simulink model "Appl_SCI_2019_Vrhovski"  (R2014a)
settings: Solver=ode45  StartTime=0.0  StopTime=1000  MaxStep=0.01  RelTol=1e-3
undefined symbols (not defined in the file): deg, H, kg, m, M, mm, N, rad, s, X, Y, Z
libraries: sm_lib x389, nesl_utility x69, simulink x7
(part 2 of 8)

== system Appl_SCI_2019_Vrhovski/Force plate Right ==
  Center of Presure : MATLAB Function  TreatAsAtomicUnit=on
  Donja ploca : Subsystem
  Gornja ploca : Subsystem
  Komponente senzora sile : Subsystem
  Senzori sile : Subsystem
  F : PMIOPort  Port=1  Side=Right
  B : PMIOPort  Port=2  Side=Left
  CoP_x : Outport
  CoP_y : Outport  Port=2
  Fz : Outport  Port=3
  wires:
  Komponente senzora sile/3(F1z) -> Center of Presure/1(Fz1)
  Komponente senzora sile/6(F2z) -> Center of Presure/2(Fz2)
  Komponente senzora sile/9(F3z) -> Center of Presure/3(Fz3)
  Komponente senzora sile/12(F4z) -> Center of Presure/4(Fz4)
  Center of Presure/1(CoP_x) -> CoP_x/1
  Center of Presure/2(CoP_y) -> CoP_y/1
  Center of Presure/3(F_suma) -> Fz/1
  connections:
  Senzori sile/RConn8 -- Komponente senzora sile/LConn4
  Senzori sile/RConn6 -- Komponente senzora sile/LConn3
  Komponente senzora sile/LConn2 -- Senzori sile/RConn4
  Senzori sile/RConn2 -- Komponente senzora sile/LConn1
  B/RConn1 -- Donja ploca/LConn1
  Gornja ploca/LConn3 -- Senzori sile/RConn5
  Senzori sile/RConn7 -- Gornja ploca/LConn4
  F/RConn1 -- Gornja ploca/RConn1
  Senzori sile/RConn3 -- Gornja ploca/LConn2
  Gornja ploca/LConn1 -- Senzori sile/RConn1
  Donja ploca/RConn4 -- Senzori sile/LConn4
  Donja ploca/RConn2 -- Senzori sile/LConn2
  Donja ploca/RConn3 -- Senzori sile/LConn3
  Donja ploca/RConn1 -- Senzori sile/LConn1

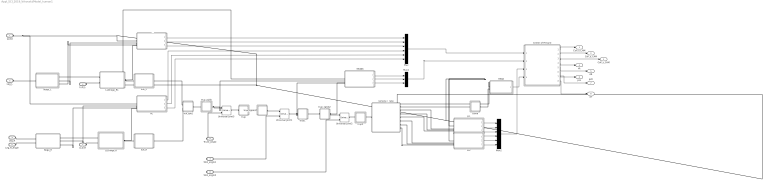
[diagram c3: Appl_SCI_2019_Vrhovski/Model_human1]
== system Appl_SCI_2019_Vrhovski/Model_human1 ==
  Center of Presure : MATLAB Function  TreatAsAtomicUnit=on
  Glava : Subsystem
  HEAD : Subsystem
  LL : Subsystem
  LL1 : Subsystem
  LL2 : Subsystem
  LLDnoge_R : Subsystem
  LLDnoge_R1 : Subsystem
  Mux : Mux  Inputs=6
  Mux1 : Mux  Inputs=3
  Mux2 : Mux  Inputs=6
  Noga_L : Subsystem
  Noga_R : Subsystem
  RL : Subsystem
  TRUNK : Subsystem
  Universal Joint1 : sm_lib/Joints/Universal Joint  SenseConstraintForce=off  SenseConstraintForceX=off  SenseConstraintForceY=off  SenseConstraintForceZ=off  SenseConstraintTorque=off  SenseConstraintTorqueX=off  SenseConstraintTorqueY=off  SenseConstraintTorqueZ=off  SenseTotalForce=off  SenseTotalForceX=off  SenseTotalForceY=off  SenseTotalForceZ=off  SenseTotalTorque=off  SenseTotalTorqueX=off  SenseTotalTorqueY=off  SenseTotalTorqueZ=off  CompositeWrenchDir=FollowerOnBase  CompositeWrenchFrame=BaseFrame  RxEquilibriumPosition=0  RxEquilibriumPositionUnits=deg  RxSpringStiffness=0  RxSpringStiffnessUnits=N*m/deg  RxDampingCoefficient=0  RxDampingCoefficientUnits=N*m/(deg/s)  RxTorqueActuationMode=ComputedTorque  RxMotionActuationMode=InputMotion  RxSensePosition=off  RxSenseVelocity=off  RxSenseAcceleration=off  RxSenseTorqueForce=off  RxPositionTargetValue=0  RxPositionTargetValueUnits=deg  RxPositionTargetSpecify=on  RxPositionTargetPriority=High  RxVelocityTargetValue=0  RxVelocityTargetValueUnits=deg/s  RxVelocityTargetSpecify=off  RxVelocityTargetPriority=High  RyEquilibriumPosition=0  RyEquilibriumPositionUnits=deg  RySpringStiffness=0  RySpringStiffnessUnits=N*m/deg  RyDampingCoefficient=0  RyDampingCoefficientUnits=N*m/(deg/s)  RyTorqueActuationMode=ComputedTorque  RyMotionActuationMode=InputMotion  RySensePosition=off  RySenseVelocity=off  RySenseAcceleration=off  RySenseTorqueForce=off  RyPositionTargetValue=0  RyPositionTargetValueUnits=deg  RyPositionTargetSpecify=off  RyPositionTargetPriority=High  RyVelocityTargetValue=0  RyVelocityTargetValueUnits=deg/s  RyVelocityTargetSpecify=off  RyVelocityTargetPriority=High  BlockFunction=simmechanics.library.joints.universal_joint
  Universal Joint2 : sm_lib/Joints/Universal Joint  SenseConstraintForce=off  SenseConstraintForceX=off  SenseConstraintForceY=off  SenseConstraintForceZ=off  SenseConstraintTorque=off  SenseConstraintTorqueX=off  SenseConstraintTorqueY=off  SenseConstraintTorqueZ=off  SenseTotalForce=off  SenseTotalForceX=off  SenseTotalForceY=off  SenseTotalForceZ=off  SenseTotalTorque=off  SenseTotalTorqueX=off  SenseTotalTorqueY=off  SenseTotalTorqueZ=off  CompositeWrenchDir=FollowerOnBase  CompositeWrenchFrame=BaseFrame  RxEquilibriumPosition=0  RxEquilibriumPositionUnits=deg  RxSpringStiffness=0  RxSpringStiffnessUnits=N*m/deg  RxDampingCoefficient=0  RxDampingCoefficientUnits=N*m/(deg/s)  RxTorqueActuationMode=ComputedTorque  RxMotionActuationMode=InputMotion  RxSensePosition=off  RxSenseVelocity=off  RxSenseAcceleration=off  RxSenseTorqueForce=off  RxPositionTargetValue=0  RxPositionTargetValueUnits=deg  RxPositionTargetSpecify=on  RxPositionTargetPriority=High  RxVelocityTargetValue=0  RxVelocityTargetValueUnits=deg/s  RxVelocityTargetSpecify=off  RxVelocityTargetPriority=High  RyEquilibriumPosition=0  RyEquilibriumPositionUnits=deg  RySpringStiffness=0  RySpringStiffnessUnits=N*m/deg  RyDampingCoefficient=0  RyDampingCoefficientUnits=N*m/(deg/s)  RyTorqueActuationMode=ComputedTorque  RyMotionActuationMode=InputMotion  RySensePosition=off  RySenseVelocity=off  RySenseAcceleration=off  RySenseTorqueForce=off  RyPositionTargetValue=0  RyPositionTargetValueUnits=deg  RyPositionTargetSpecify=off  RyPositionTargetPriority=High  RyVelocityTargetValue=0  RyVelocityTargetValueUnits=deg/s  RyVelocityTargetSpecify=off  RyVelocityTargetPriority=High  BlockFunction=simmechanics.library.joints.universal_joint
  Universal Joint5 : sm_lib/Joints/Universal Joint  SenseConstraintForce=off  SenseConstraintForceX=off  SenseConstraintForceY=off  SenseConstraintForceZ=off  SenseConstraintTorque=off  SenseConstraintTorqueX=off  SenseConstraintTorqueY=off  SenseConstraintTorqueZ=off  SenseTotalForce=off  SenseTotalForceX=off  SenseTotalForceY=off  SenseTotalForceZ=off  SenseTotalTorque=off  SenseTotalTorqueX=off  SenseTotalTorqueY=off  SenseTotalTorqueZ=off  CompositeWrenchDir=FollowerOnBase  CompositeWrenchFrame=BaseFrame  RxEquilibriumPosition=0  RxEquilibriumPositionUnits=deg  RxSpringStiffness=0  RxSpringStiffnessUnits=N*m/deg  RxDampingCoefficient=0  RxDampingCoefficientUnits=N*m/(deg/s)  RxTorqueActuationMode=ComputedTorque  RxMotionActuationMode=InputMotion  RxSensePosition=off  RxSenseVelocity=off  RxSenseAcceleration=off  RxSenseTorqueForce=off  RxPositionTargetValue=0  RxPositionTargetValueUnits=deg  RxPositionTargetSpecify=on  RxPositionTargetPriority=High  RxVelocityTargetValue=0  RxVelocityTargetValueUnits=deg/s  RxVelocityTargetSpecify=off  RxVelocityTargetPriority=High  RyEquilibriumPosition=0  RyEquilibriumPositionUnits=deg  RySpringStiffness=0  RySpringStiffnessUnits=N*m/deg  RyDampingCoefficient=0  RyDampingCoefficientUnits=N*m/(deg/s)  RyTorqueActuationMode=ComputedTorque  RyMotionActuationMode=InputMotion  RySensePosition=off  RySenseVelocity=off  RySenseAcceleration=off  RySenseTorqueForce=off  RyPositionTargetValue=0  RyPositionTargetValueUnits=deg  RyPositionTargetSpecify=off  RyPositionTargetPriority=High  RyVelocityTargetValue=0  RyVelocityTargetValueUnits=deg/s  RyVelocityTargetSpecify=off  RyVelocityTargetPriority=High  BlockFunction=simmechanics.library.joints.universal_joint
  kuk_L : Subsystem
  kuk_R : Subsystem
  kuk_spoj : Subsystem
  ramena_i_ruke : Subsystem
  trup : Subsystem
  trup1 : Subsystem
  trup2 : Subsystem
  trup_zglob : Subsystem
  trup_zglob1 : Subsystem
  trup_zglob2 : Subsystem
  world : PMIOPort  Port=1  Side=Left
  Leg_L : PMIOPort  Port=2  Side=Left
  LLD_L : PMIOPort  Port=3  Side=Left
  Leg_R : PMIOPort  Port=4  Side=Left
  LLD_R : PMIOPort  Port=5  Side=Left
  Leg_R_Angle : PMIOPort  Port=6  Side=Left
  Skol_angle1 : PMIOPort  Port=7  Side=Right
  Skol_angle2 : PMIOPort  Port=8  Side=Right
  Trunk_Angle : PMIOPort  Port=9  Side=Right
  CoP_x_CAM : Outport
  CoP_y_CAM : Outport  Port=2
  CoP_z_CAM : Outport  Port=3
  dL : Outport  Port=4
  dR : Outport  Port=5
  pzL : Outport  Port=6
  pzR : Outport  Port=7
  dT : Outport  Port=8
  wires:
  LL/1(Lxyz1) -> Mux/1
  LL/2(Lxyz2) -> Mux/2
  LL/3(Lxyz3) -> Mux/3
  RL/1(Lxyz1) -> Mux/4
  RL/2(Lxyz2) -> Mux/5
  RL/3(Lxyz3) -> Mux/6
  TRUNK/2(Txyz2) -> Mux1/2
  TRUNK/1(Txyz1) -> Mux1/1
  TRUNK/3(Txyz3) -> Mux1/3
  Mux1/1 -> Center of Presure/2(trunk_marker)
  HEAD/1(xyz) -> Center of Presure/4(head_marker)
  LL1/2(Lxyz2) -> Mux2/2
  LL1/1(Lxyz1) -> Mux2/1
  LL1/3(Lxyz3) -> Mux2/3
  LL2/3(Lxyz3) -> Mux2/6
  LL2/1(Lxyz1) -> Mux2/4
  LL2/2(Lxyz2) -> Mux2/5
  Mux2/1 -> Center of Presure/3(hand_marker)
  Center of Presure/1(CoP_x) -> CoP_x_CAM/1
  Center of Presure/2(CoP_y) -> CoP_y_CAM/1
  Center of Presure/3(CoP_z) -> CoP_z_CAM/1
  Mux/1 -> Center of Presure/1(leg_marker)
  Center of Presure/4(dL) -> dL/1
  Center of Presure/5(dR) -> dR/1
  Center of Presure/6(pzL) -> pzL/1
  Center of Presure/7(pzR) -> pzR/1
  Center of Presure/8(dT) -> dT/1
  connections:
  trup_zglob/RConn1 -- TRUNK/LConn2 -- Universal Joint5/LConn1
  Universal Joint5/RConn1 -- trup/LConn1
  kuk_spoj/LConn1 -- trup_zglob/LConn1
  LLDnoge_R/RConn1 -- RL/LConn4 -- kuk_R/LConn1
  LLD_R/RConn1 -- LLDnoge_R/LConn2
  LLD_L/RConn1 -- LLDnoge_R1/LConn2
  Leg_R/RConn1 -- Noga_R/LConn1
  Leg_R_Angle/RConn1 -- Noga_R/LConn2
  trup_zglob1/LConn1 -- trup/RConn1
  trup1/LConn1 -- TRUNK/LConn3 -- Universal Joint1/RConn1
  trup_zglob1/RConn1 -- Universal Joint1/LConn1
  trup1/RConn1 -- trup_zglob2/LConn1
  trup2/LConn1 -- Universal Joint2/RConn1
  trup_zglob2/RConn1 -- TRUNK/LConn4 -- Universal Joint2/LConn1
  Skol_angle1/RConn1 -- Universal Joint1/LConn3
  Skol_angle2/RConn1 -- Universal Joint2/LConn3
  Trunk_Angle/RConn1 -- Universal Joint5/LConn3
  kuk_spoj/RConn1 -- kuk_L/RConn1
  kuk_spoj/RConn2 -- kuk_R/RConn1
  LLDnoge_R1/RConn1 -- LL/LConn4 -- kuk_L/LConn1
  Leg_L/RConn1 -- Noga_L/LConn1
  LL/LConn2 -- Noga_L/RConn2
  Noga_L/RConn3 -- LL/LConn3
  world/RConn1 -- RL/LConn1 -- LL2/LConn1 -- LL1/LConn1 -- HEAD/LConn1 -- TRUNK/LConn1 -- LL/LConn1
  RL/LConn2 -- Noga_R/RConn2
  RL/LConn3 -- Noga_R/RConn3
  HEAD/LConn2 -- Glava/RConn1
  trup2/RConn1 -- ramena_i_ruke/LConn1
  ramena_i_ruke/RConn1 -- Glava/LConn1
  LL1/LConn2 -- ramena_i_ruke/RConn2
  LL1/LConn3 -- ramena_i_ruke/RConn3
  LL1/LConn4 -- ramena_i_ruke/RConn4
  ramena_i_ruke/RConn6 -- LL2/LConn3
  ramena_i_ruke/RConn5 -- LL2/LConn2
  ramena_i_ruke/RConn7 -- LL2/LConn4
  Noga_R/RConn1 -- LLDnoge_R/LConn1
  Noga_L/RConn1 -- LLDnoge_R1/LConn1

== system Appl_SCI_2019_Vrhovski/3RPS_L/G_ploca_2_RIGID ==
  ReferenceFrame : sm_lib/Frames and Transforms/Reference Frame  BlockFunction=simmechanics.library.frames_transforms.reference_frame
  Solid : sm_lib/Body Elements/Solid  InertiaType=Custom  Mass=5  MassUnits=kg  CenterOfMass=[-1.0925911726464245e-05 0 -4.4436244658035022]  CenterOfMassUnits=mm  MomentsOfInertia=[45540 79860 45540]  MomentsOfInertiaUnits=kg*mm^2  ProductsOfInertia=[0 -0.00010369999054466602 0]  ProductsOfInertiaUnits=kg*mm^2  DensityBased=on  Density=1000  DensityUnits=kg/(m^3)  GraphicType=FromGeometry  MarkerShape=Sphere  MarkerSize=10  MarkerSizeUnits=m  GraphicVisPropType=SimpleVisualProperties  GraphicDiffuseColor=[0.4 0.4 0.4]  GraphicSpecularColor=[0.5 0.5 0.5 1.0]  GraphicAmbientColor=[0.15 0.15 0.15 1.0]  GraphicEmissiveColor=[0.0 0.0 0.0 1.0]  GraphicShininess=75  GraphicOpacity=1  GeometryShape=Brick  RectangleSize=[1 1]  RectangleSizeUnits=m  BrickDimensions=[240 210 20]  BrickDimensionUnits=mm  CylinderRadius=120  CylinderRadiusUnits=mm  CylinderLength=20  CylinderLengthUnits=mm  SphereRadius=1  SphereRadiusUnits=m  EllipsoidRadii=[1 1 1]  EllipsoidRadiiUnits=m  ExtrusionCrossSection=[1 1; -1 1; -1 -1; 1 -1]  ExtrusionCrossSectionUnits=m  ExtrusionLength=1  ExtrusionLengthUnits=m  PolygonNumSides=3  PolygonOuterRadius=1  PolygonOuterRadiusUnits=m  ExtGeomFileType=STL  ExtGeomFileName=G_ploca_Default_sldprt.STL  ExtGeomFileUnits=mm  RevolutionCrossSection=[1 1; 1 -1; 2 -1; 2 1]  RevolutionCrossSectionUnits=m  RevolutionExtent=Full  RevolutionAngle=180  RevolutionAngleUnits=deg  BlockFunction=simmechanics.library.body_elements.solid
  Transform : sm_lib/Frames and Transforms/Rigid Transform  TranslationMethod=Cartesian  TranslationLengthUnit=mm  TranslationStandardAxis=+Z  TranslationStandardOffset=0  TranslationCartesianOffset="[-50.0000   -86.6025         -10]"  TranslationROffset=0  TranslationROffsetUnits=m  TranslationZOffset=0  TranslationZOffsetUnits=m  TranslationThetaOffset=0  TranslationThetaOffsetUnits=deg  RotationMethod=ArbitraryAxis  RotationAngleUnits=rad  RotationStandardAxis=+Z  RotationAngle=0  RotationArbitraryAxis=[0 0 0]  FollAlignAxisA=+X  BaseAlignAxisA=+Y  FollAlignAxisB=+Y  BaseAlignAxisB=+Z  BlockFunction=simmechanics.library.frames_transforms.rigid_transform
  Transform1 : sm_lib/Frames and Transforms/Rigid Transform  TranslationMethod=Cartesian  TranslationLengthUnit=mm  TranslationStandardAxis=+Z  TranslationStandardOffset=0  TranslationCartesianOffset="[-50.0000   86.6025         -10]"  TranslationROffset=0  TranslationROffsetUnits=m  TranslationZOffset=0  TranslationZOffsetUnits=m  TranslationThetaOffset=0  TranslationThetaOffsetUnits=deg  RotationMethod=ArbitraryAxis  RotationAngleUnits=rad  RotationStandardAxis=+Z  RotationAngle=0  RotationArbitraryAxis=[0 0 0]  FollAlignAxisA=+X  BaseAlignAxisA=+Y  FollAlignAxisB=+Y  BaseAlignAxisB=+Z  BlockFunction=simmechanics.library.frames_transforms.rigid_transform
  Transform2 : sm_lib/Frames and Transforms/Rigid Transform  TranslationMethod=Cartesian  TranslationLengthUnit=mm  TranslationStandardAxis=+Z  TranslationStandardOffset=0  TranslationCartesianOffset=[100 0 -10]  TranslationROffset=0  TranslationROffsetUnits=m  TranslationZOffset=0  TranslationZOffsetUnits=m  TranslationThetaOffset=0  TranslationThetaOffsetUnits=deg  RotationMethod=ArbitraryAxis  RotationAngleUnits=rad  RotationStandardAxis=+Z  RotationAngle=0  RotationArbitraryAxis=[0 0 0]  FollAlignAxisA=+X  BaseAlignAxisA=+Y  FollAlignAxisB=+Y  BaseAlignAxisB=+Z  BlockFunction=simmechanics.library.frames_transforms.rigid_transform
  Transform3 : sm_lib/Frames and Transforms/Rigid Transform  TranslationMethod=StandardAxis  TranslationLengthUnit=mm  TranslationStandardAxis=+Z  TranslationStandardOffset=10  TranslationCartesianOffset=[80.000000000002558 4.2632564145606011e-14 -32.999999999999048]  TranslationROffset=0  TranslationROffsetUnits=m  TranslationZOffset=0  TranslationZOffsetUnits=m  TranslationThetaOffset=0  TranslationThetaOffsetUnits=deg  RotationMethod=None  RotationAngleUnits=rad  RotationStandardAxis=+Z  RotationAngle=0  RotationArbitraryAxis=[0 0 0]  FollAlignAxisA=+X  BaseAlignAxisA=+Y  FollAlignAxisB=+Y  BaseAlignAxisB=+Z  BlockFunction=simmechanics.library.frames_transforms.rigid_transform
  F2 : PMIOPort  Port=1  Side=Left
  F1 : PMIOPort  Port=2  Side=Left
  F : PMIOPort  Port=3  Side=Left
  F3 : PMIOPort  Port=4  Side=Right
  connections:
  ReferenceFrame/RConn1 -- Transform/LConn1 -- Transform1/LConn1 -- Transform2/LConn1 -- Transform3/LConn1 -- Solid/RConn1
  Transform/RConn1 -- F/RConn1
  Transform1/RConn1 -- F1/RConn1
  Transform2/RConn1 -- F2/RConn1
  Transform3/RConn1 -- F3/RConn1

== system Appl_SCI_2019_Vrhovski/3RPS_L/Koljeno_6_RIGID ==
  ReferenceFrame : sm_lib/Frames and Transforms/Reference Frame  BlockFunction=simmechanics.library.frames_transforms.reference_frame
  Solid : sm_lib/Body Elements/Solid  InertiaType=Custom  Mass=1.2  MassUnits=kg  CenterOfMass=[0 94.726347166305388 0]  CenterOfMassUnits=mm  MomentsOfInertia=[342 72 342]  MomentsOfInertiaUnits=kg*mm^2  ProductsOfInertia=[0 0 0]  ProductsOfInertiaUnits=kg*mm^2  DensityBased=on  Density=1000  DensityUnits=kg/(m^3)  GraphicType=FromGeometry  MarkerShape=Sphere  MarkerSize=10  MarkerSizeUnits=m  GraphicVisPropType=SimpleVisualProperties  GraphicDiffuseColor=[0.792156862745098 0.81960784313725488 0.93333333333333335]  GraphicSpecularColor=[0.5 0.5 0.5 1.0]  GraphicAmbientColor=[0.15 0.15 0.15 1.0]  GraphicEmissiveColor=[0.0 0.0 0.0 1.0]  GraphicShininess=75  GraphicOpacity=1  GeometryShape=FromFile  RectangleSize=[1 1]  RectangleSizeUnits=m  BrickDimensions=[1 1 1]  BrickDimensionUnits=m  CylinderRadius=1  CylinderRadiusUnits=m  CylinderLength=1  CylinderLengthUnits=m  SphereRadius=1  SphereRadiusUnits=m  EllipsoidRadii=[1 1 1]  EllipsoidRadiiUnits=m  ExtrusionCrossSection=[1 1; -1 1; -1 -1; 1 -1]  ExtrusionCrossSectionUnits=m  ExtrusionLength=1  ExtrusionLengthUnits=m  PolygonNumSides=3  PolygonOuterRadius=1  PolygonOuterRadiusUnits=m  ExtGeomFileType=STL  ExtGeomFileName=E:\Fer 2\Doktorski studij\Doktorat\LLD\matlab\LLD 3RPS\PS_limb.STL  ExtGeomFileUnits=mm  RevolutionCrossSection=[1 1; 1 -1; 2 -1; 2 1]  RevolutionCrossSectionUnits=m  RevolutionExtent=Full  RevolutionAngle=180  RevolutionAngleUnits=deg  BlockFunction=simmechanics.library.body_elements.solid
  Transform : sm_lib/Frames and Transforms/Rigid Transform  TranslationMethod=Cartesian  TranslationLengthUnit=mm  TranslationStandardAxis=+Z  TranslationStandardOffset=0  TranslationCartesianOffset=[2.9560869854197764e-13 -4.9068237247312261e-13 -4.0348858674063459e-14]  TranslationROffset=0  TranslationROffsetUnits=m  TranslationZOffset=0  TranslationZOffsetUnits=m  TranslationThetaOffset=0  TranslationThetaOffsetUnits=deg  RotationMethod=ArbitraryAxis  RotationAngleUnits=rad  RotationStandardAxis=+Z  RotationAngle=2.0943951023931988  RotationArbitraryAxis=[-0.57735026918962673 -0.57735026918962595 -0.57735026918962451]  FollAlignAxisA=+X  BaseAlignAxisA=+Y  FollAlignAxisB=+Y  BaseAlignAxisB=+Z  BlockFunction=simmechanics.library.frames_transforms.rigid_transform
  Transform1 : sm_lib/Frames and Transforms/Rigid Transform  TranslationMethod=Cartesian  TranslationLengthUnit=mm  TranslationStandardAxis=+Z  TranslationStandardOffset=0  TranslationCartesianOffset=[0 162 0]  TranslationROffset=0  TranslationROffsetUnits=m  TranslationZOffset=0  TranslationZOffsetUnits=m  TranslationThetaOffset=0  TranslationThetaOffsetUnits=deg  RotationMethod=ArbitraryAxis  RotationAngleUnits=rad  RotationStandardAxis=+Z  RotationAngle=0  RotationArbitraryAxis=[0 0 0]  FollAlignAxisA=+X  BaseAlignAxisA=+Y  FollAlignAxisB=+Y  BaseAlignAxisB=+Z  BlockFunction=simmechanics.library.frames_transforms.rigid_transform
  F : PMIOPort  Port=1  Side=Left
  F1 : PMIOPort  Port=2  Side=Right
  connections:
  Solid/RConn1 -- ReferenceFrame/RConn1 -- Transform/LConn1 -- Transform1/LConn1
  Transform/RConn1 -- F/RConn1
  Transform1/RConn1 -- F1/RConn1

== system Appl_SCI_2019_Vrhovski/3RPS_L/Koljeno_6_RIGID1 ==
  ReferenceFrame : sm_lib/Frames and Transforms/Reference Frame  BlockFunction=simmechanics.library.frames_transforms.reference_frame
  Solid : sm_lib/Body Elements/Solid  InertiaType=Custom  Mass=1.2  MassUnits=kg  CenterOfMass=[0 94.726347166305388 0]  CenterOfMassUnits=mm  MomentsOfInertia=[342 72 342]  MomentsOfInertiaUnits=kg*mm^2  ProductsOfInertia=[0 0 0]  ProductsOfInertiaUnits=kg*mm^2  DensityBased=on  Density=1000  DensityUnits=kg/(m^3)  GraphicType=FromGeometry  MarkerShape=Sphere  MarkerSize=10  MarkerSizeUnits=m  GraphicVisPropType=SimpleVisualProperties  GraphicDiffuseColor=[0.792156862745098 0.81960784313725488 0.93333333333333335]  GraphicSpecularColor=[0.5 0.5 0.5 1.0]  GraphicAmbientColor=[0.15 0.15 0.15 1.0]  GraphicEmissiveColor=[0.0 0.0 0.0 1.0]  GraphicShininess=75  GraphicOpacity=1  GeometryShape=FromFile  RectangleSize=[1 1]  RectangleSizeUnits=m  BrickDimensions=[1 1 1]  BrickDimensionUnits=m  CylinderRadius=1  CylinderRadiusUnits=m  CylinderLength=1  CylinderLengthUnits=m  SphereRadius=1  SphereRadiusUnits=m  EllipsoidRadii=[1 1 1]  EllipsoidRadiiUnits=m  ExtrusionCrossSection=[1 1; -1 1; -1 -1; 1 -1]  ExtrusionCrossSectionUnits=m  ExtrusionLength=1  ExtrusionLengthUnits=m  PolygonNumSides=3  PolygonOuterRadius=1  PolygonOuterRadiusUnits=m  ExtGeomFileType=STL  ExtGeomFileName=E:\Fer 2\Doktorski studij\Doktorat\LLD\matlab\LLD 3RPS\PS_limb.STL  ExtGeomFileUnits=mm  RevolutionCrossSection=[1 1; 1 -1; 2 -1; 2 1]  RevolutionCrossSectionUnits=m  RevolutionExtent=Full  RevolutionAngle=180  RevolutionAngleUnits=deg  BlockFunction=simmechanics.library.body_elements.solid
  Transform : sm_lib/Frames and Transforms/Rigid Transform  TranslationMethod=Cartesian  TranslationLengthUnit=mm  TranslationStandardAxis=+Z  TranslationStandardOffset=0  TranslationCartesianOffset=[2.9560869854197764e-13 -4.9068237247312261e-13 -4.0348858674063459e-14]  TranslationROffset=0  TranslationROffsetUnits=m  TranslationZOffset=0  TranslationZOffsetUnits=m  TranslationThetaOffset=0  TranslationThetaOffsetUnits=deg  RotationMethod=ArbitraryAxis  RotationAngleUnits=rad  RotationStandardAxis=+Z  RotationAngle=2.0943951023931988  RotationArbitraryAxis=[-0.57735026918962673 -0.57735026918962595 -0.57735026918962451]  FollAlignAxisA=+X  BaseAlignAxisA=+Y  FollAlignAxisB=+Y  BaseAlignAxisB=+Z  BlockFunction=simmechanics.library.frames_transforms.rigid_transform
  Transform1 : sm_lib/Frames and Transforms/Rigid Transform  TranslationMethod=Cartesian  TranslationLengthUnit=mm  TranslationStandardAxis=+Z  TranslationStandardOffset=0  TranslationCartesianOffset=[0 161.99999999999997 0]  TranslationROffset=0  TranslationROffsetUnits=m  TranslationZOffset=0  TranslationZOffsetUnits=m  TranslationThetaOffset=0  TranslationThetaOffsetUnits=deg  RotationMethod=ArbitraryAxis  RotationAngleUnits=rad  RotationStandardAxis=+Z  RotationAngle=0  RotationArbitraryAxis=[0 0 0]  FollAlignAxisA=+X  BaseAlignAxisA=+Y  FollAlignAxisB=+Y  BaseAlignAxisB=+Z  BlockFunction=simmechanics.library.frames_transforms.rigid_transform
  F : PMIOPort  Port=1  Side=Left
  F1 : PMIOPort  Port=2  Side=Right
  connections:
  Transform1/RConn1 -- F1/RConn1
  Transform/RConn1 -- F/RConn1
  Solid/RConn1 -- ReferenceFrame/RConn1 -- Transform1/LConn1 -- Transform/LConn1

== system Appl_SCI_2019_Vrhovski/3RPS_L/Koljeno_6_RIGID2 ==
  ReferenceFrame : sm_lib/Frames and Transforms/Reference Frame  BlockFunction=simmechanics.library.frames_transforms.reference_frame
  Solid : sm_lib/Body Elements/Solid  InertiaType=Custom  Mass=1.2  MassUnits=kg  CenterOfMass=[0 94.726347166305388 0]  CenterOfMassUnits=mm  MomentsOfInertia=[342 72 342]  MomentsOfInertiaUnits=kg*mm^2  ProductsOfInertia=[0 0 0]  ProductsOfInertiaUnits=kg*mm^2  DensityBased=on  Density=1000  DensityUnits=kg/(m^3)  GraphicType=FromGeometry  MarkerShape=Sphere  MarkerSize=10  MarkerSizeUnits=m  GraphicVisPropType=SimpleVisualProperties  GraphicDiffuseColor=[0.792156862745098 0.81960784313725488 0.93333333333333335]  GraphicSpecularColor=[0.5 0.5 0.5 1.0]  GraphicAmbientColor=[0.15 0.15 0.15 1.0]  GraphicEmissiveColor=[0.0 0.0 0.0 1.0]  GraphicShininess=75  GraphicOpacity=1  GeometryShape=FromFile  RectangleSize=[1 1]  RectangleSizeUnits=m  BrickDimensions=[1 1 1]  BrickDimensionUnits=m  CylinderRadius=1  CylinderRadiusUnits=m  CylinderLength=1  CylinderLengthUnits=m  SphereRadius=1  SphereRadiusUnits=m  EllipsoidRadii=[1 1 1]  EllipsoidRadiiUnits=m  ExtrusionCrossSection=[1 1; -1 1; -1 -1; 1 -1]  ExtrusionCrossSectionUnits=m  ExtrusionLength=1  ExtrusionLengthUnits=m  PolygonNumSides=3  PolygonOuterRadius=1  PolygonOuterRadiusUnits=m  ExtGeomFileType=STL  ExtGeomFileName=E:\Fer 2\Doktorski studij\Doktorat\LLD\matlab\LLD 3RPS\PS_limb.STL  ExtGeomFileUnits=mm  RevolutionCrossSection=[1 1; 1 -1; 2 -1; 2 1]  RevolutionCrossSectionUnits=m  RevolutionExtent=Full  RevolutionAngle=180  RevolutionAngleUnits=deg  BlockFunction=simmechanics.library.body_elements.solid
  Transform : sm_lib/Frames and Transforms/Rigid Transform  TranslationMethod=Cartesian  TranslationLengthUnit=mm  TranslationStandardAxis=+Z  TranslationStandardOffset=0  TranslationCartesianOffset=[2.9560869854197764e-13 -4.9068237247312261e-13 -4.0348858674063459e-14]  TranslationROffset=0  TranslationROffsetUnits=m  TranslationZOffset=0  TranslationZOffsetUnits=m  TranslationThetaOffset=0  TranslationThetaOffsetUnits=deg  RotationMethod=ArbitraryAxis  RotationAngleUnits=rad  RotationStandardAxis=+Z  RotationAngle=2.0943951023931988  RotationArbitraryAxis=[-0.57735026918962673 -0.57735026918962595 -0.57735026918962451]  FollAlignAxisA=+X  BaseAlignAxisA=+Y  FollAlignAxisB=+Y  BaseAlignAxisB=+Z  BlockFunction=simmechanics.library.frames_transforms.rigid_transform
  Transform1 : sm_lib/Frames and Transforms/Rigid Transform  TranslationMethod=Cartesian  TranslationLengthUnit=mm  TranslationStandardAxis=+Z  TranslationStandardOffset=0  TranslationCartesianOffset=[0 161.99999999999997 0]  TranslationROffset=0  TranslationROffsetUnits=m  TranslationZOffset=0  TranslationZOffsetUnits=m  TranslationThetaOffset=0  TranslationThetaOffsetUnits=deg  RotationMethod=ArbitraryAxis  RotationAngleUnits=rad  RotationStandardAxis=+Z  RotationAngle=0  RotationArbitraryAxis=[0 0 0]  FollAlignAxisA=+X  BaseAlignAxisA=+Y  FollAlignAxisB=+Y  BaseAlignAxisB=+Z  BlockFunction=simmechanics.library.frames_transforms.rigid_transform
  F : PMIOPort  Port=1  Side=Left
  F1 : PMIOPort  Port=2  Side=Right
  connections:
  Transform/LConn1 -- Transform1/LConn1 -- ReferenceFrame/RConn1 -- Solid/RConn1
  Transform/RConn1 -- F/RConn1
  Transform1/RConn1 -- F1/RConn1

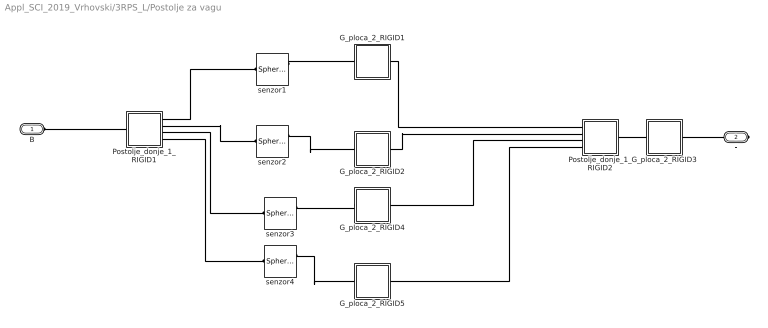
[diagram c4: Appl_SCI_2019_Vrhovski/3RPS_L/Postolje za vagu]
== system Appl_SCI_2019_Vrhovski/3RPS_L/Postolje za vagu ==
  G_ploca_2_RIGID1 : Subsystem
  G_ploca_2_RIGID2 : Subsystem
  G_ploca_2_RIGID3 : Subsystem
  G_ploca_2_RIGID4 : Subsystem
  G_ploca_2_RIGID5 : Subsystem
  Postolje_donje_1_RIGID1 : Subsystem
  Postolje_donje_1_RIGID2 : Subsystem
  senzor{1..4} (4 alike) : sm_lib/Joints/Spherical Joint  SenseConstraintForce=off  SenseConstraintForceX=off  SenseConstraintForceY=off  SenseConstraintForceZ=off  SenseConstraintTorque=off  SenseConstraintTorqueX=off  SenseConstraintTorqueY=off  SenseConstraintTorqueZ=off  SenseTotalForce=on  SenseTotalForceX=off  SenseTotalForceY=off  SenseTotalForceZ=off  SenseTotalTorque=off  SenseTotalTorqueX=off  SenseTotalTorqueY=off  SenseTotalTorqueZ=off  CompositeWrenchDir=FollowerOnBase  CompositeWrenchFrame=BaseFrame  DefPosRotationMethod=None  DefPosRotationAngleUnits=deg  DefPosRotationStandardAxis=+Z  DefPosRotationAngle=0  DefPosRotationArbitraryAxis=[0 0 1]  DefPosFollAlignAxisA=+X  DefPosBaseAlignAxisA=+Y  DefPosFollAlignAxisB=+Y  DefPosBaseAlignAxisB=+Z  EqPosRotationMethod=None  EqPosRotationAngleUnits=deg  EqPosRotationStandardAxis=+Z  EqPosRotationAngle=0  EqPosRotationArbitraryAxis=[0 0 1]  EqPosFollAlignAxisA=+X  EqPosBaseAlignAxisA=+Y  EqPosFollAlignAxisB=+Y  EqPosBaseAlignAxisB=+Z  SpringStiffness=0  SpringStiffnessUnits=m*N/rad  DampingCoefficient=0  DampingCoefficientUnits=m*s*N/rad  ActuateTorqueX=off  ActuateTorqueY=off  ActuateTorqueZ=off  ActuateTorque=off  TorqueActuationMode=NoTorque  MotionActuationMode=ComputedMotion  ActuationFrame=BaseFrame  SensePosition=off  SenseVelocityX=off  SenseVelocityY=off  SenseVelocityZ=off  SenseVelocity=off  SenseAccelerationX=off  SenseAccelerationY=off  SenseAccelerationZ=off  SenseAcceleration=off  SenseTorqueX=off  SenseTorqueY=off  SenseTorqueZ=off  SenseTorqueForce=off  SensingFrame=FollowerFrame  PositionTargetRotationMethod=None  PositionTargetRotationAngleUnits=deg  PositionTargetRotationStandardAxis=+Z  PositionTargetRotationAngle=0  PositionTargetRotationArbitraryAxis=[0 0 1]  PositionTargetFollAlignAxisA=+X  PositionTargetBaseAlignAxisA=+Y  PositionTargetFollAlignAxisB=+Y  PositionTargetBaseAlignAxisB=+Z  PositionTargetSpecify=off  PositionTargetPriority=High  VelocityTargetValue=[0 0 0]  VelocityTargetValueUnits=deg/s  VelocityTargetSpecify=off  VelocityTargetPriority=High  VelocityTargetInFollowerFrame=on  BlockFunction=simmechanics.library.joints.spherical_joint
  B : PMIOPort  Port=1  Side=Left
  F : PMIOPort  Port=2  Side=Right
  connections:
  B/RConn1 -- Postolje_donje_1_RIGID1/LConn1
  G_ploca_2_RIGID4/LConn1 -- senzor3/RConn1
  senzor2/LConn1 -- Postolje_donje_1_RIGID1/RConn2
  senzor4/LConn1 -- Postolje_donje_1_RIGID1/RConn4
  senzor4/RConn1 -- G_ploca_2_RIGID5/LConn1
  G_ploca_2_RIGID1/RConn1 -- Postolje_donje_1_RIGID2/LConn1
  G_ploca_2_RIGID2/RConn1 -- Postolje_donje_1_RIGID2/LConn2
  senzor3/LConn1 -- Postolje_donje_1_RIGID1/RConn3
  G_ploca_2_RIGID5/RConn1 -- Postolje_donje_1_RIGID2/LConn4
  G_ploca_2_RIGID3/RConn1 -- F/RConn1
  G_ploca_2_RIGID3/LConn1 -- Postolje_donje_1_RIGID2/RConn1
  G_ploca_2_RIGID4/RConn1 -- Postolje_donje_1_RIGID2/LConn3
  senzor2/RConn1 -- G_ploca_2_RIGID2/LConn1
  Postolje_donje_1_RIGID1/RConn1 -- senzor1/LConn1
  senzor1/RConn1 -- G_ploca_2_RIGID1/LConn1

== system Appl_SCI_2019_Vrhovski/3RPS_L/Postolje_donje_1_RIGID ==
  ReferenceFrame : sm_lib/Frames and Transforms/Reference Frame  BlockFunction=simmechanics.library.frames_transforms.reference_frame
  Solid : sm_lib/Body Elements/Solid  InertiaType=Custom  Mass=62.206189968539466  MassUnits=kg  CenterOfMass=[0 0 2.5]  CenterOfMassUnits=mm  MomentsOfInertia=[58000.590195722754395 58000.590195722754238 114000.2247851136613]  MomentsOfInertiaUnits=kg*mm^2  ProductsOfInertia=[0 0 0]  ProductsOfInertiaUnits=kg*mm^2  DensityBased=on  Density=10000  DensityUnits=kg/(m^3)  GraphicType=FromGeometry  MarkerShape=Sphere  MarkerSize=10  MarkerSizeUnits=m  GraphicVisPropType=SimpleVisualProperties  GraphicDiffuseColor=[0.4 0.4 0.4]  GraphicSpecularColor=[0.5 0.5 0.5 1.0]  GraphicAmbientColor=[0.15 0.15 0.15 1.0]  GraphicEmissiveColor=[0.0 0.0 0.0 1.0]  GraphicShininess=75  GraphicOpacity=1  GeometryShape=Cylinder  RectangleSize=[1 1]  RectangleSizeUnits=m  BrickDimensions=[300 180 5]  BrickDimensionUnits=mm  CylinderRadius=60  CylinderRadiusUnits=mm  CylinderLength=10  CylinderLengthUnits=mm  SphereRadius=1  SphereRadiusUnits=m  EllipsoidRadii=[1 1 1]  EllipsoidRadiiUnits=m  ExtrusionCrossSection=[1 1; -1 1; -1 -1; 1 -1]  ExtrusionCrossSectionUnits=m  ExtrusionLength=1  ExtrusionLengthUnits=m  PolygonNumSides=3  PolygonOuterRadius=1  PolygonOuterRadiusUnits=m  ExtGeomFileType=STL  ExtGeomFileName=Postolje_donje_Default_sldprt.STL  ExtGeomFileUnits=mm  RevolutionCrossSection=[1 1; 1 -1; 2 -1; 2 1]  RevolutionCrossSectionUnits=m  RevolutionExtent=Full  RevolutionAngle=180  RevolutionAngleUnits=deg  BlockFunction=simmechanics.library.body_elements.solid
  Transform : sm_lib/Frames and Transforms/Rigid Transform  TranslationMethod=Cartesian  TranslationLengthUnit=mm  TranslationStandardAxis=+Z  TranslationStandardOffset=0  TranslationCartesianOffset="[-30.0000   -51.9615         0]"  TranslationROffset=0  TranslationROffsetUnits=m  TranslationZOffset=0  TranslationZOffsetUnits=m  TranslationThetaOffset=0  TranslationThetaOffsetUnits=deg  RotationMethod=ArbitraryAxis  RotationAngleUnits=rad  RotationStandardAxis=+Z  RotationAngle=1.8234765819369776  RotationArbitraryAxis=[0.77459666924148252 0.44721359549995954 0.44721359549995798]  FollAlignAxisA=+X  BaseAlignAxisA=+Y  FollAlignAxisB=+Y  BaseAlignAxisB=+Z  BlockFunction=simmechanics.library.frames_transforms.rigid_transform
  Transform1 : sm_lib/Frames and Transforms/Rigid Transform  TranslationMethod=Cartesian  TranslationLengthUnit=mm  TranslationStandardAxis=+Z  TranslationStandardOffset=0  TranslationCartesianOffset="[ -30.0000   51.9615         0]"  TranslationROffset=0  TranslationROffsetUnits=m  TranslationZOffset=0  TranslationZOffsetUnits=m  TranslationThetaOffset=0  TranslationThetaOffsetUnits=deg  RotationMethod=ArbitraryAxis  RotationAngleUnits=rad  RotationStandardAxis=+Z  RotationAngle=2.41885840577637  RotationArbitraryAxis=[0.37796447300923008 0.65465367070797587 0.65465367070797675]  FollAlignAxisA=+X  BaseAlignAxisA=+Y  FollAlignAxisB=+Y  BaseAlignAxisB=+Z  BlockFunction=simmechanics.library.frames_transforms.rigid_transform
  Transform2 : sm_lib/Frames and Transforms/Rigid Transform  TranslationMethod=Cartesian  TranslationLengthUnit=mm  TranslationStandardAxis=+Z  TranslationStandardOffset=0  TranslationCartesianOffset="[60     0     0]"  TranslationROffset=0  TranslationROffsetUnits=m  TranslationZOffset=0  TranslationZOffsetUnits=m  TranslationThetaOffset=0  TranslationThetaOffsetUnits=deg  RotationMethod=ArbitraryAxis  RotationAngleUnits=rad  RotationStandardAxis=+Z  RotationAngle=2.0943951023931975  RotationArbitraryAxis=[0.57735026918962651 -0.57735026918962651 0.5773502691896244]  FollAlignAxisA=+X  BaseAlignAxisA=+Y  FollAlignAxisB=+Y  BaseAlignAxisB=+Z  BlockFunction=simmechanics.library.frames_transforms.rigid_transform
  F3 : PMIOPort  Port=1  Side=Left
  F2 : PMIOPort  Port=2  Side=Right
  F1 : PMIOPort  Port=3  Side=Right
  F : PMIOPort  Port=4  Side=Right
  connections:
  Transform/RConn1 -- F/RConn1
  Transform1/RConn1 -- F1/RConn1
  Transform2/RConn1 -- F2/RConn1
  Solid/RConn1 -- ReferenceFrame/RConn1 -- Transform2/LConn1 -- Transform1/LConn1 -- Transform/LConn1 -- F3/RConn1

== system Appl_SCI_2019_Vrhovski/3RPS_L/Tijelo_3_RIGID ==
  ReferenceFrame : sm_lib/Frames and Transforms/Reference Frame  BlockFunction=simmechanics.library.frames_transforms.reference_frame
  Solid : sm_lib/Body Elements/Solid  InertiaType=Custom  Mass=3.25  MassUnits=kg  CenterOfMass=[0 67.696607712724699 0]  CenterOfMassUnits=mm  MomentsOfInertia=[7450 490 7450]  MomentsOfInertiaUnits=kg*mm^2  ProductsOfInertia=[0 0 0]  ProductsOfInertiaUnits=kg*mm^2  DensityBased=on  Density=1000  DensityUnits=kg/(m^3)  GraphicType=FromGeometry  MarkerShape=Sphere  MarkerSize=10  MarkerSizeUnits=m  GraphicVisPropType=SimpleVisualProperties  GraphicDiffuseColor=[0.4 0.4 0.4]  GraphicSpecularColor=[0.5 0.5 0.5 1.0]  GraphicAmbientColor=[0.15 0.15 0.15 1.0]  GraphicEmissiveColor=[0.0 0.0 0.0 1.0]  GraphicShininess=75  GraphicOpacity=1  GeometryShape=FromFile  RectangleSize=[1 1]  RectangleSizeUnits=m  BrickDimensions=[1 1 1]  BrickDimensionUnits=m  CylinderRadius=1  CylinderRadiusUnits=m  CylinderLength=1  CylinderLengthUnits=m  SphereRadius=1  SphereRadiusUnits=m  EllipsoidRadii=[1 1 1]  EllipsoidRadiiUnits=m  ExtrusionCrossSection=[1 1; -1 1; -1 -1; 1 -1]  ExtrusionCrossSectionUnits=m  ExtrusionLength=1  ExtrusionLengthUnits=m  PolygonNumSides=3  PolygonOuterRadius=1  PolygonOuterRadiusUnits=m  ExtGeomFileType=STL  ExtGeomFileName=E:\Fer 2\Doktorski studij\Doktorat\LLD\matlab\LLD 3RPS\RP_limb.STL  ExtGeomFileUnits=mm  RevolutionCrossSection=[1 1; 1 -1; 2 -1; 2 1]  RevolutionCrossSectionUnits=m  RevolutionExtent=Full  RevolutionAngle=180  RevolutionAngleUnits=deg  BlockFunction=simmechanics.library.body_elements.solid
  Transform : sm_lib/Frames and Transforms/Rigid Transform  TranslationMethod=Cartesian  TranslationLengthUnit=mm  TranslationStandardAxis=+Z  TranslationStandardOffset=0  TranslationCartesianOffset=[0 150 0]  TranslationROffset=0  TranslationROffsetUnits=m  TranslationZOffset=0  TranslationZOffsetUnits=m  TranslationThetaOffset=0  TranslationThetaOffsetUnits=deg  RotationMethod=ArbitraryAxis  RotationAngleUnits=rad  RotationStandardAxis=+Z  RotationAngle=2.0943951023931953  RotationArbitraryAxis=[-0.57735026918962584 -0.57735026918962584 -0.57735026918962584]  FollAlignAxisA=+X  BaseAlignAxisA=+Y  FollAlignAxisB=+Y  BaseAlignAxisB=+Z  BlockFunction=simmechanics.library.frames_transforms.rigid_transform
  Transform1 : sm_lib/Frames and Transforms/Rigid Transform  TranslationMethod=Cartesian  TranslationLengthUnit=mm  TranslationStandardAxis=+Z  TranslationStandardOffset=0  TranslationCartesianOffset=[0 -10 0]  TranslationROffset=0  TranslationROffsetUnits=m  TranslationZOffset=0  TranslationZOffsetUnits=m  TranslationThetaOffset=0  TranslationThetaOffsetUnits=deg  RotationMethod=ArbitraryAxis  RotationAngleUnits=rad  RotationStandardAxis=+Z  RotationAngle=3.1415926535897905  RotationArbitraryAxis=[1 -1.4003819427637228e-30 -9.8290662577982061e-16]  FollAlignAxisA=+X  BaseAlignAxisA=+Y  FollAlignAxisB=+Y  BaseAlignAxisB=+Z  BlockFunction=simmechanics.library.frames_transforms.rigid_transform
  F1 : PMIOPort  Port=1  Side=Left
  F : PMIOPort  Port=2  Side=Right
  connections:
  Solid/RConn1 -- ReferenceFrame/RConn1 -- Transform/LConn1 -- Transform1/LConn1
  Transform/RConn1 -- F/RConn1
  Transform1/RConn1 -- F1/RConn1

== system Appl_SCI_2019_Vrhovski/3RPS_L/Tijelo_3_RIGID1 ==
  ReferenceFrame : sm_lib/Frames and Transforms/Reference Frame  BlockFunction=simmechanics.library.frames_transforms.reference_frame
  Solid : sm_lib/Body Elements/Solid  InertiaType=Custom  Mass=3.25  MassUnits=kg  CenterOfMass=[0 67.696607712724699 0]  CenterOfMassUnits=mm  MomentsOfInertia=[7450 490 7450]  MomentsOfInertiaUnits=kg*mm^2  ProductsOfInertia=[0 0 0]  ProductsOfInertiaUnits=kg*mm^2  DensityBased=on  Density=1000  DensityUnits=kg/(m^3)  GraphicType=FromGeometry  MarkerShape=Sphere  MarkerSize=10  MarkerSizeUnits=m  GraphicVisPropType=SimpleVisualProperties  GraphicDiffuseColor=[0.4 0.4 0.4]  GraphicSpecularColor=[0.5 0.5 0.5 1.0]  GraphicAmbientColor=[0.15 0.15 0.15 1.0]  GraphicEmissiveColor=[0.0 0.0 0.0 1.0]  GraphicShininess=75  GraphicOpacity=1  GeometryShape=FromFile  RectangleSize=[1 1]  RectangleSizeUnits=m  BrickDimensions=[1 1 1]  BrickDimensionUnits=m  CylinderRadius=1  CylinderRadiusUnits=m  CylinderLength=1  CylinderLengthUnits=m  SphereRadius=1  SphereRadiusUnits=m  EllipsoidRadii=[1 1 1]  EllipsoidRadiiUnits=m  ExtrusionCrossSection=[1 1; -1 1; -1 -1; 1 -1]  ExtrusionCrossSectionUnits=m  ExtrusionLength=1  ExtrusionLengthUnits=m  PolygonNumSides=3  PolygonOuterRadius=1  PolygonOuterRadiusUnits=m  ExtGeomFileType=STL  ExtGeomFileName=E:\Fer 2\Doktorski studij\Doktorat\LLD\matlab\LLD 3RPS\RP_limb.STL  ExtGeomFileUnits=mm  RevolutionCrossSection=[1 1; 1 -1; 2 -1; 2 1]  RevolutionCrossSectionUnits=m  RevolutionExtent=Full  RevolutionAngle=180  RevolutionAngleUnits=deg  BlockFunction=simmechanics.library.body_elements.solid
  Transform : sm_lib/Frames and Transforms/Rigid Transform  TranslationMethod=Cartesian  TranslationLengthUnit=mm  TranslationStandardAxis=+Z  TranslationStandardOffset=0  TranslationCartesianOffset=[0 150 0]  TranslationROffset=0  TranslationROffsetUnits=m  TranslationZOffset=0  TranslationZOffsetUnits=m  TranslationThetaOffset=0  TranslationThetaOffsetUnits=deg  RotationMethod=ArbitraryAxis  RotationAngleUnits=rad  RotationStandardAxis=+Z  RotationAngle=2.0943951023931953  RotationArbitraryAxis=[-0.57735026918962584 -0.57735026918962584 -0.57735026918962584]  FollAlignAxisA=+X  BaseAlignAxisA=+Y  FollAlignAxisB=+Y  BaseAlignAxisB=+Z  BlockFunction=simmechanics.library.frames_transforms.rigid_transform
  Transform1 : sm_lib/Frames and Transforms/Rigid Transform  TranslationMethod=Cartesian  TranslationLengthUnit=mm  TranslationStandardAxis=+Z  TranslationStandardOffset=0  TranslationCartesianOffset=[0 -10 0]  TranslationROffset=0  TranslationROffsetUnits=m  TranslationZOffset=0  TranslationZOffsetUnits=m  TranslationThetaOffset=0  TranslationThetaOffsetUnits=deg  RotationMethod=ArbitraryAxis  RotationAngleUnits=rad  RotationStandardAxis=+Z  RotationAngle=3.1415926535897905  RotationArbitraryAxis=[1 -1.4003819427637228e-30 -9.8290662577982061e-16]  FollAlignAxisA=+X  BaseAlignAxisA=+Y  FollAlignAxisB=+Y  BaseAlignAxisB=+Z  BlockFunction=simmechanics.library.frames_transforms.rigid_transform
  F1 : PMIOPort  Port=1  Side=Left
  F : PMIOPort  Port=2  Side=Right
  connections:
  Transform1/RConn1 -- F1/RConn1
  Transform/RConn1 -- F/RConn1
  ReferenceFrame/RConn1 -- Solid/RConn1 -- Transform1/LConn1 -- Transform/LConn1

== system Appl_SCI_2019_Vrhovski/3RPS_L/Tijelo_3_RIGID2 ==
  ReferenceFrame : sm_lib/Frames and Transforms/Reference Frame  BlockFunction=simmechanics.library.frames_transforms.reference_frame
  Solid : sm_lib/Body Elements/Solid  InertiaType=Custom  Mass=3.25  MassUnits=kg  CenterOfMass=[0 67.696607712724699 0]  CenterOfMassUnits=mm  MomentsOfInertia=[7450 490 7450]  MomentsOfInertiaUnits=kg*mm^2  ProductsOfInertia=[0 0 0]  ProductsOfInertiaUnits=kg*mm^2  DensityBased=on  Density=1000  DensityUnits=kg/(m^3)  GraphicType=FromGeometry  MarkerShape=Sphere  MarkerSize=10  MarkerSizeUnits=m  GraphicVisPropType=SimpleVisualProperties  GraphicDiffuseColor=[0.4 0.4 0.4]  GraphicSpecularColor=[0.5 0.5 0.5 1.0]  GraphicAmbientColor=[0.15 0.15 0.15 1.0]  GraphicEmissiveColor=[0.0 0.0 0.0 1.0]  GraphicShininess=75  GraphicOpacity=1  GeometryShape=FromFile  RectangleSize=[1 1]  RectangleSizeUnits=m  BrickDimensions=[1 1 1]  BrickDimensionUnits=m  CylinderRadius=1  CylinderRadiusUnits=m  CylinderLength=1  CylinderLengthUnits=m  SphereRadius=1  SphereRadiusUnits=m  EllipsoidRadii=[1 1 1]  EllipsoidRadiiUnits=m  ExtrusionCrossSection=[1 1; -1 1; -1 -1; 1 -1]  ExtrusionCrossSectionUnits=m  ExtrusionLength=1  ExtrusionLengthUnits=m  PolygonNumSides=3  PolygonOuterRadius=1  PolygonOuterRadiusUnits=m  ExtGeomFileType=STL  ExtGeomFileName=E:\Fer 2\Doktorski studij\Doktorat\LLD\matlab\LLD 3RPS\RP_limb.STL  ExtGeomFileUnits=mm  RevolutionCrossSection=[1 1; 1 -1; 2 -1; 2 1]  RevolutionCrossSectionUnits=m  RevolutionExtent=Full  RevolutionAngle=180  RevolutionAngleUnits=deg  BlockFunction=simmechanics.library.body_elements.solid
  Transform : sm_lib/Frames and Transforms/Rigid Transform  TranslationMethod=Cartesian  TranslationLengthUnit=mm  TranslationStandardAxis=+Z  TranslationStandardOffset=0  TranslationCartesianOffset=[0 150 0]  TranslationROffset=0  TranslationROffsetUnits=m  TranslationZOffset=0  TranslationZOffsetUnits=m  TranslationThetaOffset=0  TranslationThetaOffsetUnits=deg  RotationMethod=ArbitraryAxis  RotationAngleUnits=rad  RotationStandardAxis=+Z  RotationAngle=2.0943951023931953  RotationArbitraryAxis=[-0.57735026918962584 -0.57735026918962584 -0.57735026918962584]  FollAlignAxisA=+X  BaseAlignAxisA=+Y  FollAlignAxisB=+Y  BaseAlignAxisB=+Z  BlockFunction=simmechanics.library.frames_transforms.rigid_transform
  Transform1 : sm_lib/Frames and Transforms/Rigid Transform  TranslationMethod=Cartesian  TranslationLengthUnit=mm  TranslationStandardAxis=+Z  TranslationStandardOffset=0  TranslationCartesianOffset=[0 -10 0]  TranslationROffset=0  TranslationROffsetUnits=m  TranslationZOffset=0  TranslationZOffsetUnits=m  TranslationThetaOffset=0  TranslationThetaOffsetUnits=deg  RotationMethod=ArbitraryAxis  RotationAngleUnits=rad  RotationStandardAxis=+Z  RotationAngle=3.1415926535897905  RotationArbitraryAxis=[1 -1.4003819427637228e-30 -9.8290662577982061e-16]  FollAlignAxisA=+X  BaseAlignAxisA=+Y  FollAlignAxisB=+Y  BaseAlignAxisB=+Z  BlockFunction=simmechanics.library.frames_transforms.rigid_transform
  F1 : PMIOPort  Port=1  Side=Left
  F : PMIOPort  Port=2  Side=Right
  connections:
  Transform/LConn1 -- Transform1/LConn1 -- Solid/RConn1 -- ReferenceFrame/RConn1
  Transform/RConn1 -- F/RConn1
  Transform1/RConn1 -- F1/RConn1

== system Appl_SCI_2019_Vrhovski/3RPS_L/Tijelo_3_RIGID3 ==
  ReferenceFrame : sm_lib/Frames and Transforms/Reference Frame  BlockFunction=simmechanics.library.frames_transforms.reference_frame
  Solid : sm_lib/Body Elements/Solid  InertiaType=Custom  Mass=3.25  MassUnits=kg  CenterOfMass=[0 67.696607712724699 0]  CenterOfMassUnits=mm  MomentsOfInertia=[7450 490 7450]  MomentsOfInertiaUnits=kg*mm^2  ProductsOfInertia=[0 0 0]  ProductsOfInertiaUnits=kg*mm^2  DensityBased=on  Density=1000  DensityUnits=kg/(m^3)  GraphicType=FromGeometry  MarkerShape=Sphere  MarkerSize=10  MarkerSizeUnits=m  GraphicVisPropType=SimpleVisualProperties  GraphicDiffuseColor=[0.4 0.4 0.4]  GraphicSpecularColor=[0.5 0.5 0.5 1.0]  GraphicAmbientColor=[0.15 0.15 0.15 1.0]  GraphicEmissiveColor=[0.0 0.0 0.0 1.0]  GraphicShininess=75  GraphicOpacity=1  GeometryShape=Cylinder  RectangleSize=[1 1]  RectangleSizeUnits=m  BrickDimensions=[1 1 1]  BrickDimensionUnits=m  CylinderRadius=15  CylinderRadiusUnits=mm  CylinderLength=280  CylinderLengthUnits=mm  SphereRadius=1  SphereRadiusUnits=m  EllipsoidRadii=[1 1 1]  EllipsoidRadiiUnits=m  ExtrusionCrossSection=[1 1; -1 1; -1 -1; 1 -1]  ExtrusionCrossSectionUnits=m  ExtrusionLength=1  ExtrusionLengthUnits=m  PolygonNumSides=3  PolygonOuterRadius=1  PolygonOuterRadiusUnits=m  ExtGeomFileType=STL  ExtGeomFileName=Tijelo_Default_sldprt.STL  ExtGeomFileUnits=mm  RevolutionCrossSection=[1 1; 1 -1; 2 -1; 2 1]  RevolutionCrossSectionUnits=m  RevolutionExtent=Full  RevolutionAngle=180  RevolutionAngleUnits=deg  BlockFunction=simmechanics.library.body_elements.solid
  Transform : sm_lib/Frames and Transforms/Rigid Transform  TranslationMethod=StandardAxis  TranslationLengthUnit=mm  TranslationStandardAxis=-Z  TranslationStandardOffset=13.29  TranslationCartesianOffset=[0 10 0]  TranslationROffset=0  TranslationROffsetUnits=m  TranslationZOffset=0  TranslationZOffsetUnits=m  TranslationThetaOffset=0  TranslationThetaOffsetUnits=deg  RotationMethod=None  RotationAngleUnits=rad  RotationStandardAxis=+Z  RotationAngle=2.0943951023931953  RotationArbitraryAxis=[-0.57735026918962584 -0.57735026918962584 -0.57735026918962584]  FollAlignAxisA=+X  BaseAlignAxisA=+Y  FollAlignAxisB=+Y  BaseAlignAxisB=+Z  BlockFunction=simmechanics.library.frames_transforms.rigid_transform
  Transform1 : sm_lib/Frames and Transforms/Rigid Transform  TranslationMethod=None  TranslationLengthUnit=mm  TranslationStandardAxis=+Z  TranslationStandardOffset=0  TranslationCartesianOffset=[0 100 0]  TranslationROffset=0  TranslationROffsetUnits=m  TranslationZOffset=0  TranslationZOffsetUnits=m  TranslationThetaOffset=0  TranslationThetaOffsetUnits=deg  RotationMethod=None  RotationAngleUnits=rad  RotationStandardAxis=+Z  RotationAngle=3.1415926535897905  RotationArbitraryAxis=[1 -1.4003819427637228e-30 -9.8290662577982061e-16]  FollAlignAxisA=+X  BaseAlignAxisA=+Y  FollAlignAxisB=+Y  BaseAlignAxisB=+Z  BlockFunction=simmechanics.library.frames_transforms.rigid_transform
  F1 : PMIOPort  Port=1  Side=Left
  F : PMIOPort  Port=2  Side=Right
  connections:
  Transform1/RConn1 -- F1/RConn1
  Transform/RConn1 -- F/RConn1
  Transform1/LConn1 -- Transform/LConn1 -- ReferenceFrame/RConn1 -- Solid/RConn1

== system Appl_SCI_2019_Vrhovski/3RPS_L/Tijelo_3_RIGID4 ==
  ReferenceFrame : sm_lib/Frames and Transforms/Reference Frame  BlockFunction=simmechanics.library.frames_transforms.reference_frame
  Solid : sm_lib/Body Elements/Solid  InertiaType=Custom  Mass=3.25  MassUnits=kg  CenterOfMass=[0 67.696607712724699 0]  CenterOfMassUnits=mm  MomentsOfInertia=[7450 490 7450]  MomentsOfInertiaUnits=kg*mm^2  ProductsOfInertia=[0 0 0]  ProductsOfInertiaUnits=kg*mm^2  DensityBased=on  Density=1000  DensityUnits=kg/(m^3)  GraphicType=FromGeometry  MarkerShape=Sphere  MarkerSize=10  MarkerSizeUnits=m  GraphicVisPropType=SimpleVisualProperties  GraphicDiffuseColor=[0.4 0.4 0.4]  GraphicSpecularColor=[0.5 0.5 0.5 1.0]  GraphicAmbientColor=[0.15 0.15 0.15 1.0]  GraphicEmissiveColor=[0.0 0.0 0.0 1.0]  GraphicShininess=75  GraphicOpacity=1  GeometryShape=Cylinder  RectangleSize=[1 1]  RectangleSizeUnits=m  BrickDimensions=[1 1 1]  BrickDimensionUnits=m  CylinderRadius=15  CylinderRadiusUnits=mm  CylinderLength=280  CylinderLengthUnits=mm  SphereRadius=1  SphereRadiusUnits=m  EllipsoidRadii=[1 1 1]  EllipsoidRadiiUnits=m  ExtrusionCrossSection=[1 1; -1 1; -1 -1; 1 -1]  ExtrusionCrossSectionUnits=m  ExtrusionLength=1  ExtrusionLengthUnits=m  PolygonNumSides=3  PolygonOuterRadius=1  PolygonOuterRadiusUnits=m  ExtGeomFileType=STL  ExtGeomFileName=Tijelo_Default_sldprt.STL  ExtGeomFileUnits=mm  RevolutionCrossSection=[1 1; 1 -1; 2 -1; 2 1]  RevolutionCrossSectionUnits=m  RevolutionExtent=Full  RevolutionAngle=180  RevolutionAngleUnits=deg  BlockFunction=simmechanics.library.body_elements.solid
  Transform : sm_lib/Frames and Transforms/Rigid Transform  TranslationMethod=StandardAxis  TranslationLengthUnit=mm  TranslationStandardAxis=-Z  TranslationStandardOffset=13.29  TranslationCartesianOffset=[0 10 0]  TranslationROffset=0  TranslationROffsetUnits=m  TranslationZOffset=0  TranslationZOffsetUnits=m  TranslationThetaOffset=0  TranslationThetaOffsetUnits=deg  RotationMethod=None  RotationAngleUnits=rad  RotationStandardAxis=+Z  RotationAngle=2.0943951023931953  RotationArbitraryAxis=[-0.57735026918962584 -0.57735026918962584 -0.57735026918962584]  FollAlignAxisA=+X  BaseAlignAxisA=+Y  FollAlignAxisB=+Y  BaseAlignAxisB=+Z  BlockFunction=simmechanics.library.frames_transforms.rigid_transform
  Transform1 : sm_lib/Frames and Transforms/Rigid Transform  TranslationMethod=None  TranslationLengthUnit=mm  TranslationStandardAxis=+Z  TranslationStandardOffset=0  TranslationCartesianOffset=[0 100 0]  TranslationROffset=0  TranslationROffsetUnits=m  TranslationZOffset=0  TranslationZOffsetUnits=m  TranslationThetaOffset=0  TranslationThetaOffsetUnits=deg  RotationMethod=None  RotationAngleUnits=rad  RotationStandardAxis=+Z  RotationAngle=3.1415926535897905  RotationArbitraryAxis=[1 -1.4003819427637228e-30 -9.8290662577982061e-16]  FollAlignAxisA=+X  BaseAlignAxisA=+Y  FollAlignAxisB=+Y  BaseAlignAxisB=+Z  BlockFunction=simmechanics.library.frames_transforms.rigid_transform
  F1 : PMIOPort  Port=1  Side=Left
  F : PMIOPort  Port=2  Side=Right
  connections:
  ReferenceFrame/RConn1 -- Solid/RConn1 -- Transform1/LConn1 -- Transform/LConn1
  Transform/RConn1 -- F/RConn1
  Transform1/RConn1 -- F1/RConn1
